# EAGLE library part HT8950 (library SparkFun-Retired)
Holtek voice modulator IC, COM-10574 Retired: No prod ID (PN 5207)
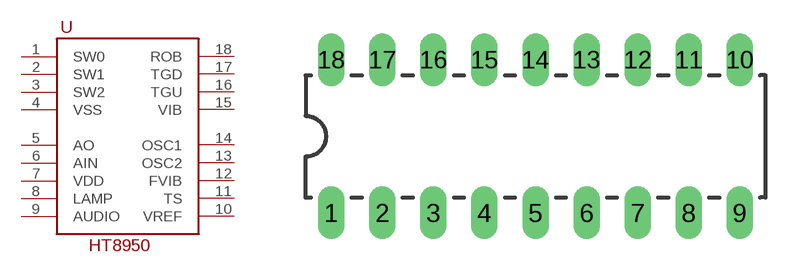
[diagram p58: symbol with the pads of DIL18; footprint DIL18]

Designator prefix -

## HT8950  [DIL18]
1  SW0
2  SW1
3  SW2
4  VSS
5  AO
6  AIN
7  VDD
8  LAMP
9  AUDIO
10  VREF
11  TS
12  FVIB
13  OSC2
14  OSC1
15  VIB
16  TGU
17  TGD
18  ROB

## Footprint DIL18 (pad centres in mm)
Dual In Line Package
drill 0.813 long: 1 -10.16,-3.81; 2 -7.62,-3.81; 3 -5.08,-3.81; 4 -2.54,-3.81; 5 0,-3.81; 6 2.54,-3.81; 7 5.08,-3.81; 8 7.62,-3.81; 9 10.16,-3.81; 10 10.16,3.81; 11 7.62,3.81; 12 5.08,3.81; 13 2.54,3.81; 14 0,3.81; 15 -2.54,3.81; 16 -5.08,3.81; 17 -7.62,3.81; 18 -10.16,3.81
